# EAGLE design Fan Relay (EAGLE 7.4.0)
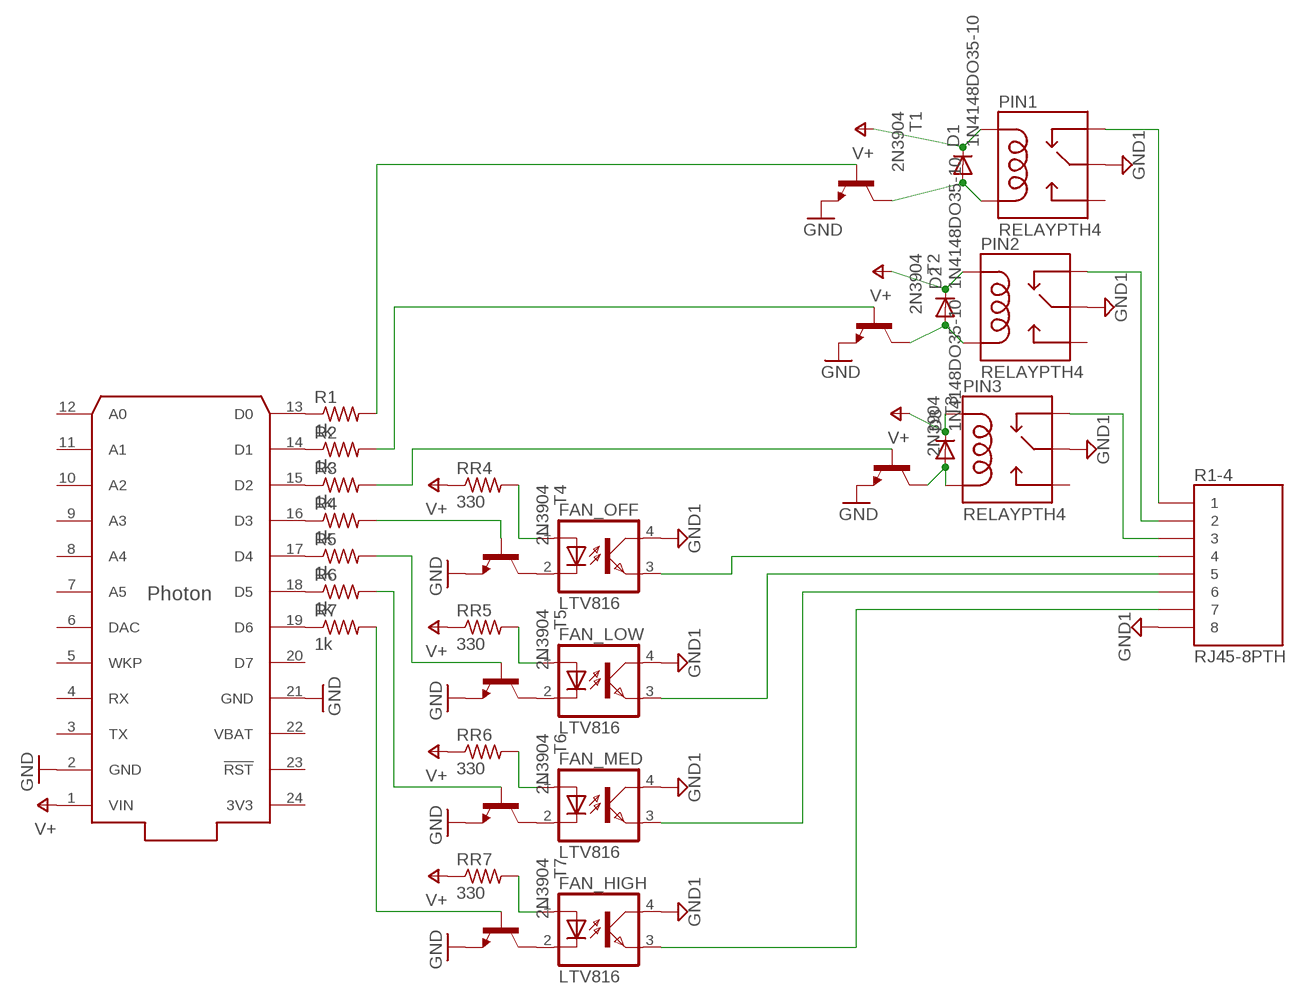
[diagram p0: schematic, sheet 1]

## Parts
D1  1N4148DO35-10  [DO35-10]
D2  1N4148DO35-10  [DO35-10]
D3  1N4148DO35-10  [DO35-10]
FAN_HIGH  LTV816  [DIL04]
FAN_LOW  LTV816  [DIL04]
FAN_MED  LTV816  [DIL04]
FAN_OFF  LTV816  [DIL04]
PHOTON  PHOTON_WITH_HEADERS  [PHOTON]
PIN1  RELAYPTH4  [RELAY-JZC]
PIN2  RELAYPTH4  [RELAY-JZC]
PIN3  RELAYPTH4  [RELAY-JZC]
R1  1k  R-US_0204/7  [0204/7]
R1-4  RJ45-8PTH  [RJ45-8]
R2  1k  R-US_0204/7  [0204/7]
R3  1k  R-US_0204/7  [0204/7]
R4  1k  R-US_0204/7  [0204/7]
R5  1k  R-US_0204/7  [0204/7]
R6  1k  R-US_0204/7  [0204/7]
R7  1k  R-US_0204/7  [0204/7]
RR4  330  R-US_0204/7  [0204/7]
RR5  330  R-US_0204/7  [0204/7]
RR6  330  R-US_0204/7  [0204/7]
RR7  330  R-US_0204/7  [0204/7]
T1  2N3904  [TO92]
T2  2N3904  [TO92]
T3  2N3904  [TO92]
T4  2N3904  [TO92]
T5  2N3904  [TO92]
T6  2N3904  [TO92]
T7  2N3904  [TO92]

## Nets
GND: PHOTON.2(GND) PHOTON.21(GND) T1.3(E) T2.3(E) T3.3(E) T4.3(E) T5.3(E) T6.3(E) T7.3(E)
GND1: FAN_HIGH.4(COL) FAN_LOW.4(COL) FAN_MED.4(COL) FAN_OFF.4(COL) PIN1.4(MAIN) PIN2.4(MAIN) PIN3.4(MAIN) R1-4.8
N$1: D1.A PIN1.1(COIL2) T1.1(C)
N$2: D2.A PIN2.1(COIL2) T2.1(C)
N$3: D3.A PIN3.1(COIL2) T3.1(C)
N$4: R1.2 T1.2(B)
N$5: R2.2 T2.2(B)
N$6: R3.2 T3.2(B)
N$7: FAN_OFF.2(C) T4.1(C)
N$8: PIN1.2(NC) R1-4.1
N$9: FAN_LOW.2(C) T5.1(C)
N$10: FAN_MED.2(C) T6.1(C)
N$11: FAN_HIGH.2(C) T7.1(C)
N$12: PIN2.2(NC) R1-4.2
N$13: PIN3.2(NC) R1-4.3
N$14: FAN_OFF.3(EMIT) R1-4.4
N$15: FAN_LOW.3(EMIT) R1-4.5
N$16: FAN_MED.3(EMIT) R1-4.6
N$17: FAN_HIGH.3(EMIT) R1-4.7
N$18: R4.2 T4.2(B)
N$19: R5.2 T5.2(B)
N$20: R6.2 T6.2(B)
N$21: R7.2 T7.2(B)
N$22: FAN_OFF.1(A) RR4.2
N$23: FAN_LOW.1(A) RR5.2
N$24: FAN_MED.1(A) RR6.2
N$25: FAN_HIGH.1(A) RR7.2
N$26: PHOTON.13(D0) R1.1
N$27: PHOTON.14(D1) R2.1
N$28: PHOTON.15(D2) R3.1
N$29: PHOTON.16(D3) R4.1
N$30: PHOTON.17(D4) R5.1
N$31: PHOTON.18(D5) R6.1
N$32: PHOTON.19(D6) R7.1
V+: D1.C D2.C D3.C PHOTON.1(VIN) PIN1.5(COIL1) PIN2.5(COIL1) PIN3.5(COIL1) RR4.1 RR5.1 RR6.1 RR7.1
Unconnected: PHOTON.3(TX) PHOTON.4(RX) PHOTON.5(WKP) PHOTON.6(DAC) PHOTON.7(A5) PHOTON.8(A4) PHOTON.9(A3) PHOTON.10(A2) PHOTON.11(A1) PHOTON.12(A0) PHOTON.20(D7) PHOTON.23(!RST) PIN1.3(NO) PIN2.3(NO) PIN3.3(NO)

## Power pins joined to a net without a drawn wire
3V3: PHOTON.24(3V3)
VBAT: PHOTON.22(VBAT)

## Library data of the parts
D1-D3 = diode:1N4148: DIODE
FAN_HIGH FAN_LOW FAN_MED FAN_OFF = optocoupler:LTV816: OPTO COUPLER Source: LITEON, LTV816.pdf; OC_FARNELL: unknown; OC_NEWARK: unknown
PHOTON = Spark:PHOTON
PIN1-PIN3 = Spark:RELAY: SPDT relay (COM-00101)
R1-R7 RR4-RR7 = rcl:R-US_: RESISTOR, American symbol
R1-4 = SparkFun-Connectors:RJ45-8: RJ45 Jack Simple RJ45, 8-pin connection - connector for common Cat5, Cat5e, and Cat6 Ethernet cables. Footprint not yet proven in production. Connector sku is PRT-00643; Breakout PCB sku is BOB-00716.
T1-T7 = transistor:2N3904: NPN TRANSISTOR

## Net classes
0 default: width 0.305 mm, drill 0.508 mm, clearance 0.254 mm

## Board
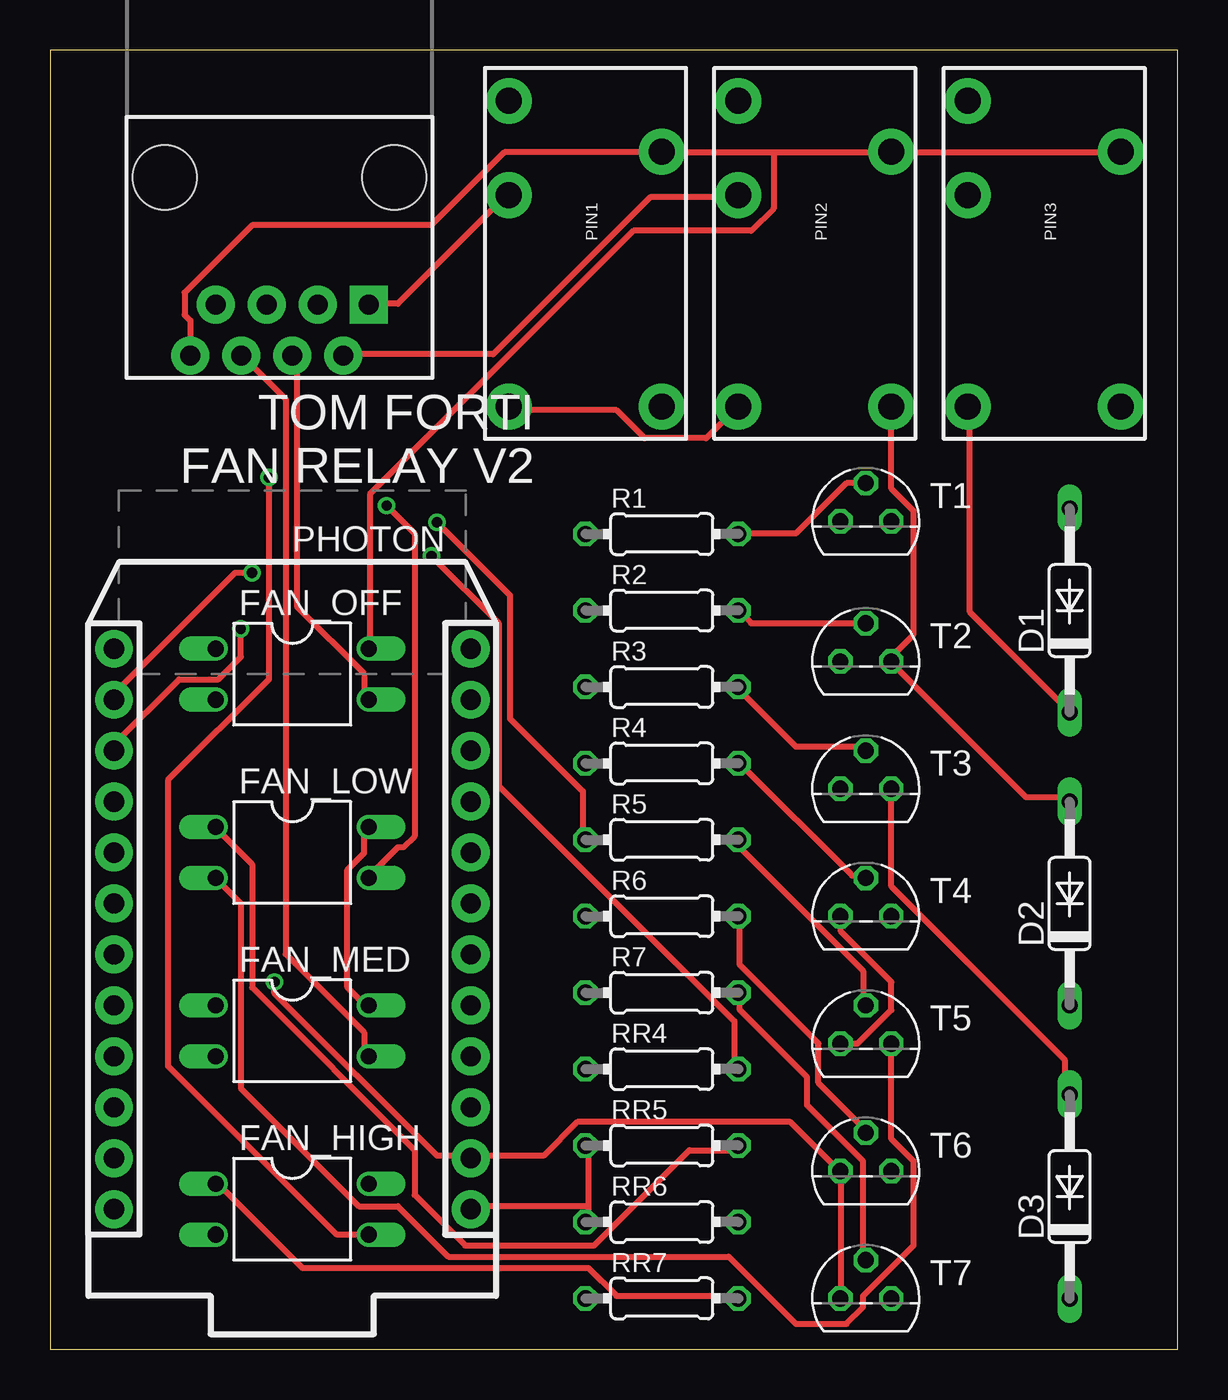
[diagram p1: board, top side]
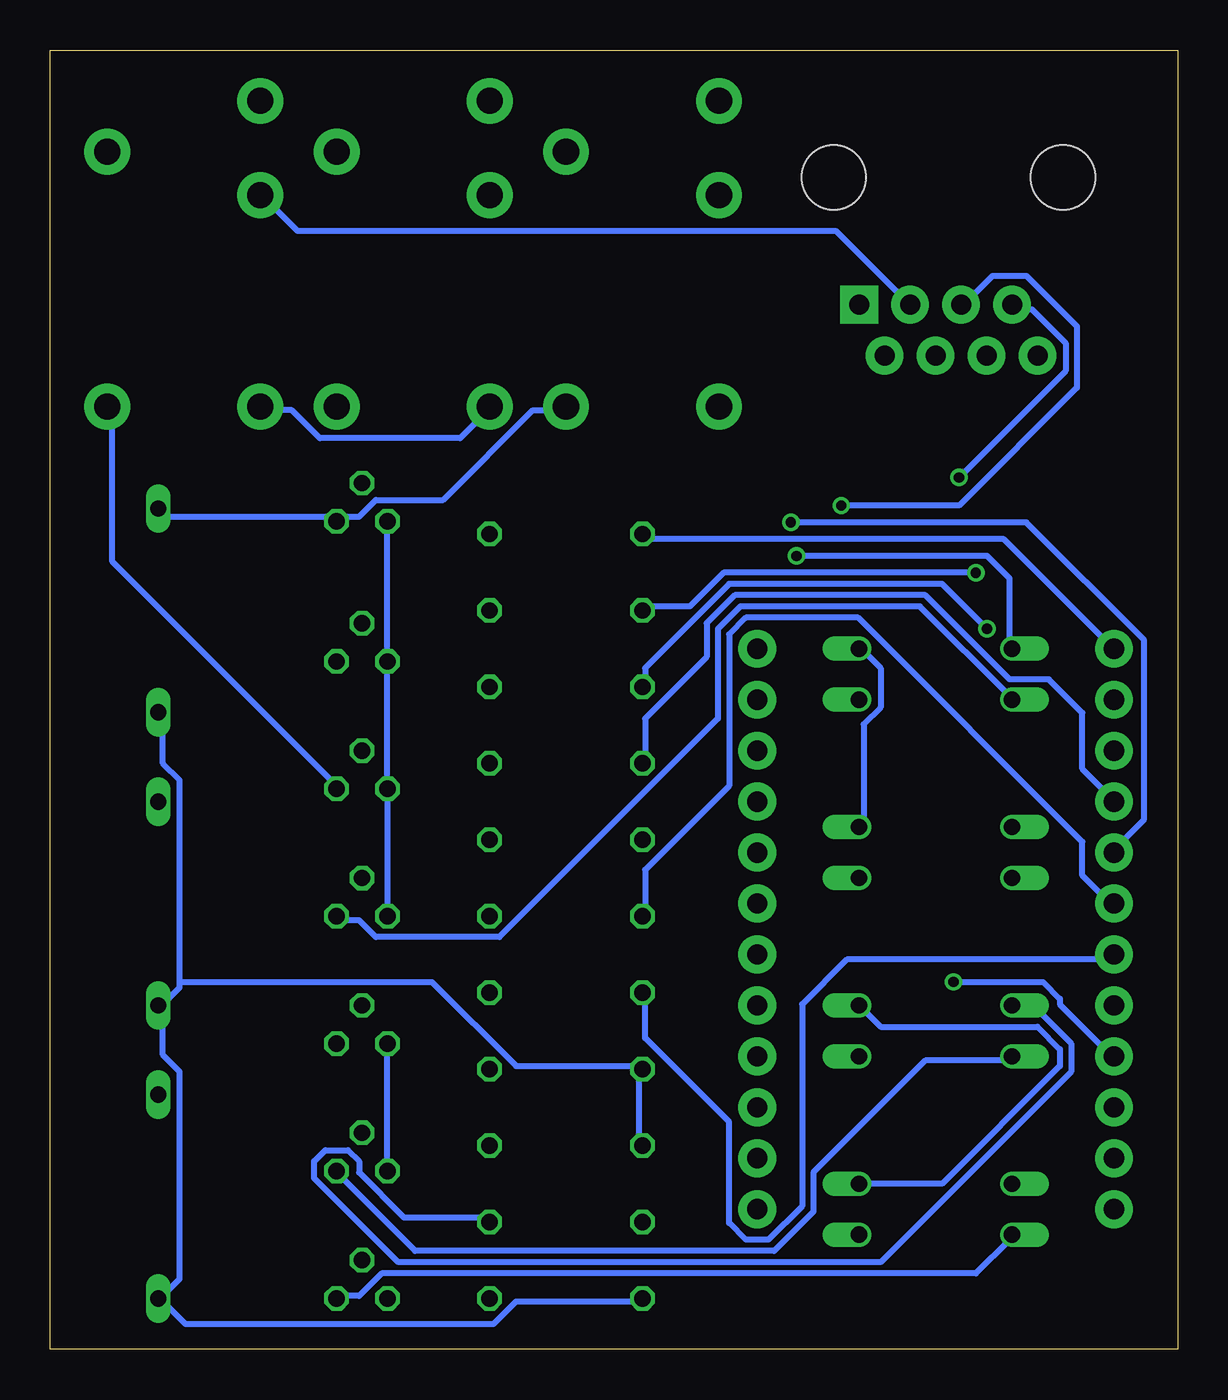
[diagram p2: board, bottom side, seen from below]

Size 56.19 x 64.76 mm. Coordinates in mm from the lower left corner, seen from the top.
Outline: 0,0 56.19,0 56.19,64.76 0,64.76 0,0
Copper layers (1*16): Top 0.0356mm / dielectric 1.5011mm / Bottom 0.0356mm
Design rules "LaenPCBOrder": minimum track width 6mil, minimum drill 13mil, track to track 6mil, track to pad 6mil, pad to pad 6mil, via to via 6mil, smd to smd 6mil, copper to edge 15mil, drill to drill 6mil, minimum pad ring 7mil, minimum via ring 7mil, stop-mask expansion 3mil, vias tented up to drill 0mil, thermal gap 10mil

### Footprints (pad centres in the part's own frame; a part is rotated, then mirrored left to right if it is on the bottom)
DO35-10 = drill 0.813 long: A 5.08,0; C -5.08,0
DIL04 = drill 0.813 offset: 1 -1.27,-3.81; 2 1.27,-3.81; 3 1.27,3.81; 4 -1.27,3.81
PHOTON = drill 1.016 pad 1.88: 1 1.27,32.258; 2 1.27,29.718; 3 1.27,27.178; 4 1.27,24.638; 5 1.27,22.098; 6 1.27,19.558; 7 1.27,17.018; 8 1.27,14.478; 9 1.27,11.938; 10 1.27,9.398; 11 1.27,6.858; 12 1.27,4.318; 13 19.05,4.318; 14 19.05,6.858; 15 19.05,9.398; 16 19.05,11.938; 17 19.05,14.478; 18 19.05,17.018; 19 19.05,19.558; 20 19.05,22.098; 21 19.05,24.638; 22 19.05,27.178; 23 19.05,29.718; 24 19.05,32.258
RELAY-JZC = drill 1.3 pad 2.286: 1 3.81,-8.89; 2 -3.81,1.651; 3 -3.81,6.35; 4 3.81,3.81; 5 -3.81,-8.89
0204/7 = drill 0.813 octagon: 1 -3.81,0; 2 3.81,0
RJ45-8 = drill 1 pad 1.88 square: 1 -4.445,6.35 | drill 1 pad 1.88: 2 -3.175,8.89; 3 -1.905,6.35; 4 -0.635,8.89; 5 0.635,6.35; 6 1.905,8.89; 7 3.175,6.35; 8 4.445,8.89 | hole 3.2: -5.715,0; 5.715,0
TO92 = drill 0.813 octagon: 1 1.27,0; 2 0,1.905; 3 -1.27,0

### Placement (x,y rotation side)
D1  50.8,36.83 90 top
D2  50.8,22.22 90 top
D3  50.8,7.62 90 top
FAN_HIGH  12.06,6.98 270 top
FAN_LOW  12.06,24.77 270 top
FAN_MED  12.06,15.88 270 top
FAN_OFF  12.06,33.66 270 top
PHOTON  22.23,39.24 180 top
PIN1  26.67,55.88 0 top
PIN2  38.1,55.88 0 top
PIN3  49.53,55.88 0 top
R1  30.48,40.64 0 top
R1-4  11.43,58.42 180 top
R2  30.48,36.83 0 top
R3  30.48,33.02 0 top
R4  30.48,29.21 0 top
R5  30.48,25.4 0 top
R6  30.48,21.59 0 top
R7  30.48,17.78 0 top
RR4  30.48,13.97 0 top
RR5  30.48,10.16 0 top
RR6  30.48,6.35 0 top
RR7  30.48,2.54 0 top
T1  40.64,41.28 0 top
T2  40.64,34.29 0 top
T3  40.64,27.94 0 top
T4  40.64,21.59 0 top
T5  40.64,15.24 0 top
T6  40.64,8.89 0 top
T7  40.64,2.54 0 top

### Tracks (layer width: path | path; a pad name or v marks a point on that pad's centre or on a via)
GND  (via drill 0.51)
  Top 0.305: T7.3 39.4,2.67 39.4,8.81 T6.3 39.12,9.09 36.88,11.33 26.26,11.33 24.59,9.65 20.95,9.65 | v11.18,18.31 11.18,17.75 19.28,9.65 20.95,9.65 | 20.95,9.65 PHOTON.2 | T5.3 40.23,15.24 41.91,16.92 41.91,18.31 39.4,20.83 39.4,21.39 T4.3
  Bottom 0.305: T4.3 39.4,21.67 39.4,27.81 T3.3 39.4,28.09 39.4,34.24 T2.3 39.4,34.52 39.4,41.22 T1.3 | T5.3 39.4,15.24 39.4,9.09 T6.3 | v11.18,18.31 6.71,18.31 5.87,17.47 5.87,17.2 3.35,14.68 PHOTON.21
GND1
  Top 0.305: FAN_LOW.4 15.65,25.86 15.65,24.74 14.81,23.9 14.81,18.03 15.65,17.2 FAN_MED.4 | R1-4.8 6.99,51.28 6.71,51.56 6.71,52.68 10.06,56.03 19,56.03 22.63,59.67 30.45,59.67 PIN1.4 30.73,59.67 36.04,59.67 | 36.04,59.67 41.91,59.67 | 41.91,59.67 53.09,59.67 PIN3.4 | 41.91,59.67 PIN2.4 | 36.04,59.67 36.04,56.87 34.92,55.75 29.06,55.75 15.93,42.62 15.93,35.08 FAN_OFF.4
  Bottom 0.305: FAN_LOW.4 15.65,26.14 15.65,31.17 14.81,32 14.81,33.96 15.65,34.8 FAN_OFF.4 | FAN_HIGH.4 11.73,8.26 5.87,14.12 5.87,14.96 6.99,16.08 14.81,16.08 FAN_MED.4
N$1
  Bottom 0.305: 41.91,41.5 50.29,41.5 50.57,41.78 D1.A | 41.91,41.5 40.79,41.5 39.95,42.34 36.6,42.34 32.13,46.81 30.73,46.81 PIN1.1 | 41.91,41.5 T1.1
N$2
  Top 0.305: D2.A 50.57,27.53 48.62,27.53 41.91,34.24 T2.1 41.91,34.52 43.03,35.64 43.03,41.78 41.91,42.9 PIN2.1
N$3
  Top 0.305: T3.1 41.91,23.06 50.57,14.4 50.57,12.72 D3.A
  Bottom 0.305: PIN3.1 53.09,46.81 53.09,39.27 41.91,28.09 T3.1
N$4
  Top 0.305: T1.2 39.67,43.18 37.16,40.67 34.37,40.67 R1.2
N$5
  Top 0.305: T2.2 34.92,36.2 R2.2
N$6
  Top 0.305: T3.2 40.51,30.05 37.16,30.05 34.37,32.84 R3.2
N$7
  Bottom 0.305: T4.1 41.91,21.39 40.79,21.39 39.95,20.55 33.81,20.55 22.91,31.45 22.91,35.92 21.79,37.03 12.85,37.03 8.38,32.56 FAN_OFF.2
N$8
  Top 0.305: R1-4.1 15.93,52.12 17.32,52.12 22.63,57.43 PIN1.2
N$9
  Top 0.305: T5.1 41.91,10.49 43.03,9.37 43.03,5.18 40.51,2.67 40.51,2.11 39.67,1.27 37.16,1.27 33.81,4.62 19.84,4.62 17.32,7.14 15.37,7.14 9.5,13 9.5,22.22 8.38,23.34 FAN_LOW.2
N$10
  Bottom 0.305: T6.1 41.91,8.81 38,4.9 20.12,4.9 18.16,6.86 18.16,8.81 12.57,14.4 8.38,14.4 FAN_MED.2
N$11
  Bottom 0.305: T7.1 41.91,2.67 40.79,2.67 39.67,3.79 10.06,3.79 8.38,5.46 FAN_HIGH.2
N$12
  Top 0.305: R1-4.2 14.81,49.61 22.07,49.61 29.9,57.43 34.09,57.43 PIN2.2
N$13
  Bottom 0.305: R1-4.3 13.41,52.12 17.04,55.75 43.87,55.75 45.54,57.43 PIN3.2
N$14
  Top 0.305: FAN_OFF.3 15.65,32.56 15.65,33.68 12.29,37.03 12.29,49.33 R1-4.4
N$15  (via drill 0.51)
  Top 0.305: v16.76,42.06 18.16,40.67 18.16,25.58 17.6,25.02 17.32,25.02 15.93,23.62 FAN_LOW.3
  Bottom 0.305: v16.76,42.06 10.9,42.06 5.03,47.93 5.03,51 7.54,53.52 9.22,53.52 10.62,52.12 R1-4.5
N$16
  Top 0.305: FAN_MED.3 15.65,14.68 15.65,15.8 11.73,19.71 11.73,47.37 9.78,49.33 R1-4.6
N$17  (via drill 0.51)
  Top 0.305: v10.9,43.46 10.9,33.4 5.87,28.37 5.87,14.12 14.25,5.74 15.65,5.74 FAN_HIGH.3
  Bottom 0.305: v10.9,43.46 5.59,48.77 5.59,50.17 7.26,51.84 8.1,51.84 R1-4.7
N$18
  Top 0.305: T4.2 40.51,23.62 39.95,23.62 34.37,29.21 R4.2
N$19
  Top 0.305: T5.2 40.51,17.2 40.51,18.87 34.09,25.3 R5.2
N$20
  Top 0.305: R6.2 34.37,21.39 34.37,19.15 38.28,15.24 38.28,13.28 40.51,11.05 T6.2
N$21
  Top 0.305: R7.2 34.37,17.75 34.37,16.92 37.72,13.56 37.72,12.17 40.51,9.37 40.51,4.62 T7.2
N$22  (via drill 0.51)
  Top 0.305: v19,39.55 22.35,36.2 22.35,28.09 34.09,16.36 34.09,14.12 RR4.2
  Bottom 0.305: v19,39.55 9.5,39.55 8.38,38.43 8.38,35.08 FAN_OFF.1
N$23
  Top 0.305: RR5.2 34.09,9.93 31.85,9.93 27.1,5.18 20.68,5.18 18.16,7.7 18.16,9.93 10.06,18.03 10.06,24.18 8.38,25.86 FAN_LOW.1
N$24
  Bottom 0.305: RR6.2 34.37,6.58 38.56,6.58 40.79,8.81 40.79,9.37 41.35,9.93 42.47,9.93 43.03,9.37 43.03,8.53 38.84,4.34 14.81,4.34 5.31,13.84 5.31,15.24 6.99,16.92 8.1,16.92 FAN_MED.1
N$25
  Top 0.305: RR7.2 34.09,2.67 28.22,2.67 26.82,4.06 12.57,4.06 8.38,8.26 FAN_HIGH.1
N$26
  Bottom 0.305: R1.1 26.54,40.39 8.66,40.39 3.35,35.08 PHOTON.13
N$27  (via drill 0.51)
  Top 0.305: v10.06,38.71 9.22,38.71 3.07,32.56 PHOTON.14
  Bottom 0.305: v10.06,38.71 22.63,38.71 24.31,37.03 26.54,37.03 R2.1
N$28  (via drill 0.51)
  Top 0.305: v9.5,35.92 9.5,34.52 8.38,33.4 6.43,33.4 3.07,30.05 PHOTON.15
  Bottom 0.305: v9.5,35.92 11.73,38.15 22.35,38.15 26.54,33.96 26.54,33.12 R3.1
N$29
  Bottom 0.305: R4.1 26.54,29.21 26.54,31.45 23.47,34.52 23.47,36.2 22.07,37.59 12.57,37.59 8.38,33.4 6.43,33.4 4.75,31.72 4.75,28.93 3.35,27.53 PHOTON.16
N$30  (via drill 0.51)
  Top 0.305: v19.28,41.22 22.91,37.59 22.91,31.45 26.54,27.81 26.54,25.58 R5.1
  Bottom 0.305: v19.28,41.22 7.54,41.22 1.68,35.36 1.68,26.42 3.07,25.02 PHOTON.17
N$31
  Bottom 0.305: R6.1 26.54,21.67 26.54,23.9 22.35,28.09 22.35,35.64 21.51,36.47 15.93,36.47 4.75,25.3 4.75,23.62 3.35,22.22 PHOTON.18
N$32
  Bottom 0.305: R7.1 26.54,17.75 26.54,15.52 22.35,11.33 22.35,6.3 21.51,5.46 20.4,5.46 18.72,7.14 18.72,17.2 16.48,19.43 3.35,19.43 PHOTON.19
V+
  Top 0.305: PIN1.5 22.91,46.81 28.22,46.81 29.62,45.42 32.69,45.42 34.09,46.81 PIN2.5 | 26.82,7.14 26.82,9.93 RR5.1 | 26.82,7.14 26.82,6.58 RR6.1 | 26.82,7.14 20.95,7.14 PHOTON.1 | PIN3.5 45.82,46.81 45.82,36.75 50.57,32 D1.C
  Bottom 0.305: PIN3.5 45.54,46.81 44.15,46.81 42.75,45.42 35.76,45.42 34.37,46.81 PIN2.5 | RR5.1 26.82,10.21 26.82,13.84 RR4.1 26.82,14.12 32.97,14.12 37.16,18.31 49.73,18.31 | RR7.1 26.82,2.39 32.97,2.39 34.09,1.27 49.45,1.27 50.57,2.39 D3.C 50.57,2.67 49.73,3.5 49.73,13.84 50.57,14.68 50.57,16.92 D2.C 50.57,17.2 49.73,18.03 49.73,18.31 | 49.73,18.31 49.73,28.37 50.57,29.21 50.57,31.72 D1.C

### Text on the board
tPlace: TOM FORTI / FAN RELAY V2

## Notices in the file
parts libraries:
SparkFun-Connectors: Licensing: CC v3.0 Share-Alike You are welcome to use this library for commercial purposes.
